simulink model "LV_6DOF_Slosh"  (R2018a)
settings: Solver=FixedStepAuto  StartTime=0.0  StopTime=489.8  FixedStep=0.0002  MaxStep=0.0001  RelTol=2e-6  EnableMultiTasking=on
InitFcn:
  | init
StopFcn:
  | pl
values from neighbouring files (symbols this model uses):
  accel = [97.3083,0,0]    [init.m]
  AcNoise = 0.1    [init.m]
  BBrcs = [82, 0.0, +3.375]    [init.m]
  Cdelay = 0.005    [init.m]
  Cza1 = FCS_Gains_Stg1(:, 5)    [init.m]
  d2r = pi/180    (= 0.0174532925199)    [init.m]    (also in pl.m; LQR_Design.m)
  Euler_0 = [90, 89.98, 0]*d2r    [init.m]
  fairing_mass = 1047.7*kg2slug    (= 71.7904994)    [init.m]
  Ie1 = 28.17    [init.m]
  Ie2 = 258.74    [init.m]
  Islosh = 1    [init.m]
  Isp = 65    [init.m]
  Ixxpr = Mass_Props(:,2)    [init.m]
  Ixypr = Mass_Props(:,5)    [init.m]
  Ixzpr = Mass_Props(:,6)    [init.m]
  Iyypr = Mass_Props(:,3)    [init.m]
  Iyzpr = Mass_Props(:,7)    [init.m]
  Izzpr = Mass_Props(:,4)    [init.m]
  Jdir = zeros(3,nt)    [init.m]
  JJ1 = Commands_2(:,2)    [init.m]
  JJ2 = Commands_2(:,3)    [init.m]
  JJ3 = Commands_2(:,4)    [init.m]
  Jloc = Jdir    [init.m]
  K_estim1 = FCS_Gains_Stg1(:,21)    [init.m]
  Kl_p1 = FCS_Gains_Stg1(:,12)    [init.m]
  Kl_phi1 = FCS_Gains_Stg1(:,11)    [init.m]
  Km_alfa1 = FCS_Gains_Stg1(:, 8)    [init.m]
  Km_alfin = FCS_Gains_Stg1(:,10)    [init.m]
  Km_q1 = FCS_Gains_Stg1(:, 7)    [init.m]
  Km_q2 = FCS_Gains_Stg2(:,5)    [init.m]
  Km_thet1 = FCS_Gains_Stg1(:, 6)    [init.m]
  Km_thet2 = FCS_Gains_Stg2(:,4)    [init.m]
  Km_thin1 = FCS_Gains_Stg1(:, 9)    [init.m]
  Km_thin2 = FCS_Gains_Stg2(:,6)    [init.m]
  Kmix2 = [ 0,   -1,    0;          0,    0,   -1]    [init.m]
  Kml1_1 = ee*FCS_Gains_Stg1(:,18)    [init.m]
  Kml2_1 = ee*FCS_Gains_Stg1(:,19)    [init.m]
  Kml2_2 = ee*FCS_Gains_Stg2(:,10)    [init.m]
  Kn_beta1 = FCS_Gains_Stg1(:,15)    [init.m]
  Kn_betin = FCS_Gains_Stg1(:,17)    [init.m]
  Kn_psi1 = FCS_Gains_Stg1(:,13)    [init.m]
  Kn_psi2 = FCS_Gains_Stg2(:,7)    [init.m]
  Kn_psin1 = FCS_Gains_Stg1(:,16)    [init.m]
  Kn_psin2 = FCS_Gains_Stg2(:,9)    [init.m]
  Kn_r1 = FCS_Gains_Stg1(:,14)    [init.m]
  Kn_r2 = FCS_Gains_Stg2(:,8)    [init.m]
  Le1 = 1.203    [init.m]
  Le2 = 2.892    [init.m]
  Massgn1 = ee*FCS_Gains_Stg1(:,2)    [init.m]
  Massgn2 = ee*FCS_Gains_Stg2(:,2)    [init.m]
  mdot1 = 2.5058    [init.m]
  mdot2 = 2.5058    [init.m]
  me1 = 9.325    [init.m]
  me2 = 13.927    [init.m]
  mrc = [x_ref, y_ref, z_ref]    [init.m]
  Msfue = Slosh(:,3)    [init.m]
  Mslox = Slosh(:,2)    [init.m]
  msspr = Mass_Props(:,1)    [init.m]
  Mvsls = Slosh(:,1)    [init.m]
  post_sep_wait = 4    [init.m]
  pre_sep_wait = 4    [init.m]
  Qbar1 = FCS_Gains_Stg1(:, 4)    [init.m]
  qtc1 = interp1(timi2(1:iend),Commands_2(1:iend, 9),timi2,'linear','extrap')    [init.m]
  qtc2 = interp1(timi2(1:iend),Commands_2(1:iend,10),timi2,'linear','extrap')    [init.m]
  qtc3 = interp1(timi2(1:iend),Commands_2(1:iend,11),timi2,'linear','extrap')    [init.m]
  qtc4 = interp1(timi2(1:iend),Commands_2(1:iend,12),timi2,'linear','extrap')    [init.m]
  r2d = 1/d2r    (= 57.2957795131)    [init.m]    (also in pl.m; LQR_Design.m)
  RBrcs = [82, +3.375, 0.0]    [init.m]
  Rfuel = Slosh(:,11)    [init.m]
  Rlox = Slosh(:,10)    [init.m]
  s1_dry_mass = 445.4969    [init.m]
  s1_init_prop_mass = 3.8002e+03    (= 3800.2)    [init.m]
  s2_dry_mass = 175.9451    [init.m]
  s2_init_prop_mass = 801.7606    [init.m]
  sp = 7.52    [init.m]
  Sref = 44.4146    [init.m]
  stage_to_fairing_sep_time = 34.7    [init.m]
  T3b = 176.6    [init.m]
  TBrcs = [82, 0.0, -3.375]    [init.m]
  thpnd = 15    [init.m]
  timi2 = Commands_2(:,1)    [init.m]
  TqLoad = 1    [init.m]
  tvc10 = [Xgmb2, 0.0,  0.0]    [init.m]
  tvc2 = [Xgmb1,  1.0202,  -2.4638]    [init.m]
  tvc3 = [Xgmb1, -1.0202,  -2.4638]    [init.m]
  tvc4 = [Xgmb1, -2.4638,  -1.0202]    [init.m]
  tvc5 = [Xgmb1, -2.4638,   1.0202]    [init.m]
  tvc6 = [Xgmb1, -1.0202,   2.4638]    [init.m]
  tvc7 = [Xgmb1,  1.0202,   2.4638]    [init.m]
  tvc8 = [Xgmb1,  2.4638,   1.0202]    [init.m]
  tvc9 = [Xgmb1,  0.0,      0.0]    [init.m]
  velpnd = 3    [init.m]
  Vrelgn1 = FCS_Gains_Stg1(:, 3)    [init.m]
  Vrelgn2 = FCS_Gains_Stg2(:,3)    [init.m]
  W_lowp1 = FCS_Gains_Stg1(:,22)    [init.m]
  W_nfilt1 = FCS_Gains_Stg1(:,20)    [init.m]
  Xcgpr = Mass_Props(:,8)    [init.m]
  Xfuel = Slosh(:,9)    [init.m]
  Xgmb1 = 10.7062    [init.m]
  Xgmb2 = 82.538    [init.m]
  Xlox = Slosh(:,8)    [init.m]
  Ycgpr = Mass_Props(:,9)    [init.m]
  Zcgpr = Mass_Props(:,10)    [init.m]
  Ztfue = Slosh(:,7)    [init.m]
  Ztlox = Slosh(:,6)    [init.m]
undefined symbols (not defined in the file or in its folder): Cl, Cl2, Cm, Cm2, Cn, Cn2, Continuous, cosd, CX, CX2, CY, CY2, CZ, CZ2, Dryden, Earth, F, ft, Isp1, Isp2, km, Kmix1, LBrcs, Light, MIL, q, r, sigbuilder_block, sind, STD, tvc1, WGS84
libraries: sharedutil x28, Actuator_Lib x18, simulink x4, aerolibasang x3, aerolibwind2 x3, sharedtransform x3, aerolibobsolete x2, aerolibconvert2 x2, aerolibatmos2 x1, aerolibadyn x1, aerolibutil x1
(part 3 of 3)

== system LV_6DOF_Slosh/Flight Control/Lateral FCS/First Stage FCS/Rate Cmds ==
  " " : Terminator
  Demux : Demux  Outputs=3
  Roll Rate Cmd : DiscretePulseGenerator  PulseType=Time based  Amplitude=10*d2r  Period=830  PhaseDelay=3.1  SampleTime=0.0002
  Sum1 : Sum  Inputs=-+|
  Transfer Fcn : TransferFcn  Denominator=[1 1]
  Pcm : Outport
  Rcm : Outport  Port=2
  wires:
  Demux/2 -> " "/1
  Demux/1 -> Sum1/2
  Sum1/1 -> Pcm/1
  [Gyros] -> Demux/1
  Demux/3 -> Rcm/1
  Roll Rate Cmd/1 -> Transfer Fcn/1
  Transfer Fcn/1 -> Sum1/1

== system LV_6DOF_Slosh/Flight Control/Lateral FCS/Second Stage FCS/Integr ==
  in : Inport
  Ground2 : Ground
  Switch : Switch  Criteria=u2 > Threshold
  int3 : Integrator
  ou : Outport
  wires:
  Ground2/1 -> Switch/3
  [s2_startup] -> Switch/2
  Switch/1 -> int3/1
  in/1 -> Switch/1
  int3/1 -> ou/1

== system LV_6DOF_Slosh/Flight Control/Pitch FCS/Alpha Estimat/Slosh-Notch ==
  note: Slosh Notch Filter
  In : Inport
  Ground : Ground
  Int1 : Integrator
  K_estim1 : Lookup  InputValues=Vrelgn1  Table=K_estim1
  Notch Filter : Subsystem
  Product1 : Product
  Switch1 : Switch  Criteria=u2 > Threshold
  Switch3 : Switch  Threshold=0.5
  Out : Outport
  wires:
  Product1/1 -> Int1/1
  Int1/1 -> Out/1
  [V0] -> K_estim1/1
  [Wnf] -> Switch3/2
  In/1 -> Switch1/3, Switch3/3
  Notch Filter/1(y) -> Switch3/1
  K_estim1/1 -> Product1/1
  [stage_sep] -> Switch1/2
  Ground/1 -> Switch1/1
  Switch1/1 -> Notch Filter/1(u)
  Switch3/1 -> Product1/2

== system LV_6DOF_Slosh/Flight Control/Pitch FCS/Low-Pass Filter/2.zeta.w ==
  in : Inport
  2.zet.w : Gain  Gain=1.25
  Product1 : Product
  ou : Outport
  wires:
  2.zet.w/1 -> Product1/1
  Product1/1 -> ou/1
  in/1 -> Product1/2
  [Wlp] -> 2.zet.w/1

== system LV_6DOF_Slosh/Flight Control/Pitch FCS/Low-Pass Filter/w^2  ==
  in : Inport
  Product : Product
  Product1 : Product
  ou : Outport
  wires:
  [Wlp] -> Product/1, Product/2
  Product/1 -> Product1/1
  Product1/1 -> ou/1
  in/1 -> Product1/2

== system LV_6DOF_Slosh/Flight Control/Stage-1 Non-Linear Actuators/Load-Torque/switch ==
  in : Inport
  Ground : Ground
  Ground1 : Ground
  Switch : Switch  Criteria=u2 > Threshold  Threshold=0.5
  Switch1 : Switch  Criteria=u2 > Threshold
  Torque Load Switch : Constant  Value=TqLoad
  ou : Outport
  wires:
  Torque Load Switch/1 -> Switch/2
  in/1 -> Switch/1
  Ground/1 -> Switch/3
  [s1_shutdown] -> Switch1/2
  Switch/1 -> Switch1/3
  Ground1/1 -> Switch1/1
  Switch1/1 -> ou/1

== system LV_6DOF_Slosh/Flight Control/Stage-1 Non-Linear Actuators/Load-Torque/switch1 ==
  in : Inport
  Ground : Ground
  Ground1 : Ground
  Switch : Switch  Criteria=u2 > Threshold  Threshold=0.5
  Switch1 : Switch  Criteria=u2 > Threshold
  Torque Load Switch : Constant  Value=TqLoad
  ou : Outport
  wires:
  Torque Load Switch/1 -> Switch/2
  in/1 -> Switch/1
  Ground/1 -> Switch/3
  [s1_shutdown] -> Switch1/2
  Switch/1 -> Switch1/3
  Ground1/1 -> Switch1/1
  Switch1/1 -> ou/1

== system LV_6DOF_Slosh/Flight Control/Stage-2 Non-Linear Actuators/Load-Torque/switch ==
  in : Inport
  Ground : Ground
  Ground1 : Ground
  Switch : Switch  Criteria=u2 > Threshold  Threshold=0.5
  Switch1 : Switch  Criteria=u2 > Threshold
  Torque Load Switch : Constant  Value=TqLoad
  ou : Outport
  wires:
  Torque Load Switch/1 -> Switch/2
  in/1 -> Switch/1
  Ground/1 -> Switch/3
  Switch1/1 -> ou/1
  Switch/1 -> Switch1/1
  Ground1/1 -> Switch1/3
  [s2_startup] -> Switch1/2

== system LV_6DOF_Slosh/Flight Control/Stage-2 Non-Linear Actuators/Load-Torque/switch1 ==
  in : Inport
  Ground : Ground
  Ground1 : Ground
  Switch : Switch  Criteria=u2 > Threshold  Threshold=0.5
  Switch1 : Switch  Criteria=u2 > Threshold
  Torque Load Switch : Constant  Value=TqLoad
  ou : Outport
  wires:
  Torque Load Switch/1 -> Switch/2
  in/1 -> Switch/1
  Ground/1 -> Switch/3
  Switch1/1 -> ou/1
  Switch/1 -> Switch1/1
  Ground1/1 -> Switch1/3
  [s2_startup] -> Switch1/2

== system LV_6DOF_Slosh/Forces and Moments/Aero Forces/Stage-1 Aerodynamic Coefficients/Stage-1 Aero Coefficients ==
  note: Stage-1 Aero
  albet : Inport
  Mach : Inport  Port=2
  Alpha Lookup : PreLookup  BreakpointsData=Alfa1  BeginIndexSearchUsingPreviousIndexResult=on  ExtrapMethod=Linear
  Beta Lookup : PreLookup  BreakpointsData=Beta1  BeginIndexSearchUsingPreviousIndexResult=on  ExtrapMethod=Linear
  CX : Interpolation_n-D  NumberOfTableDimensions=3  Table=CX  RemoveProtectionIndex=on
  CY : Interpolation_n-D  NumberOfTableDimensions=3  Table=CY  RemoveProtectionIndex=on
  CZ : Interpolation_n-D  NumberOfTableDimensions=3  Table=CZ  RemoveProtectionIndex=on
  Cl : Interpolation_n-D  NumberOfTableDimensions=3  Table=Cl  RemoveProtectionIndex=on  OutDataTypeStr=double
  Cm : Interpolation_n-D  NumberOfTableDimensions=3  Table=Cm  RemoveProtectionIndex=on
  Cn : Interpolation_n-D  NumberOfTableDimensions=3  Table=Cn  RemoveProtectionIndex=on
  Demux : Demux  Outputs=2
  Mach Lookup : PreLookup  BreakpointsData=Mach1  BeginIndexSearchUsingPreviousIndexResult=on  ExtrapMethod=Linear
  Mux1 : Mux  Inputs=6
  Coeff : Outport  InitialOutput=0
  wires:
  Mux1/1 -> Coeff/1
  Mach/1 -> Mach Lookup/1
  albet/1 -> Demux/1
  Demux/2 -> Beta Lookup/1
  Beta Lookup/2 -> CZ/6, Cl/6, Cn/6, Cm/6, CY/6, CX/6
  Beta Lookup/1 -> CY/5, CZ/5, Cl/5, Cn/5, Cm/5, CX/5
  Mach Lookup/2 -> CX/4, CZ/4, Cl/4, Cn/4, Cm/4, CY/4
  Mach Lookup/1 -> CX/3, CZ/3, Cl/3, Cn/3, Cm/3, CY/3
  Alpha Lookup/2 -> Cn/2, Cm/2, Cl/2, CZ/2, CY/2, CX/2
  Alpha Lookup/1 -> CZ/1, Cl/1, Cn/1, Cm/1, CY/1, CX/1
  Cn/1 -> Mux1/6
  Cm/1 -> Mux1/5
  Cl/1 -> Mux1/4
  CZ/1 -> Mux1/3
  CY/1 -> Mux1/2
  CX/1 -> Mux1/1
  Demux/1 -> Alpha Lookup/1

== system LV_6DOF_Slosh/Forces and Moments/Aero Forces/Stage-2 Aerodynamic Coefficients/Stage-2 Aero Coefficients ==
  note: Stage-2 Aero
  albet : Inport
  Mach : Inport  Port=2
  Alpha Lookup : PreLookup  BreakpointsData=Alfa2  BeginIndexSearchUsingPreviousIndexResult=on  ExtrapMethod=Linear
  Beta Lookup : PreLookup  BreakpointsData=Beta2  BeginIndexSearchUsingPreviousIndexResult=on  ExtrapMethod=Linear
  CX2 : Interpolation_n-D  NumberOfTableDimensions=3  Table=CX2  RemoveProtectionIndex=on
  CY2 : Interpolation_n-D  NumberOfTableDimensions=3  Table=CY2  RemoveProtectionIndex=on
  CZ2 : Interpolation_n-D  NumberOfTableDimensions=3  Table=CZ2  RemoveProtectionIndex=on
  Cl2 : Interpolation_n-D  NumberOfTableDimensions=3  Table=Cl2  RemoveProtectionIndex=on  OutDataTypeStr=double
  Cm2 : Interpolation_n-D  NumberOfTableDimensions=3  Table=Cm2  RemoveProtectionIndex=on
  Cn2 : Interpolation_n-D  NumberOfTableDimensions=3  Table=Cn2  RemoveProtectionIndex=on
  Demux : Demux  Outputs=2
  Mach Lookup : PreLookup  BreakpointsData=Mach2  BeginIndexSearchUsingPreviousIndexResult=on  ExtrapMethod=Linear
  Mux1 : Mux  Inputs=6
  Coeff : Outport  InitialOutput=0
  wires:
  Mux1/1 -> Coeff/1
  Mach/1 -> Mach Lookup/1
  albet/1 -> Demux/1
  Demux/2 -> Beta Lookup/1
  Beta Lookup/2 -> CZ2/6, Cl2/6, Cn2/6, Cm2/6, CY2/6, CX2/6
  Beta Lookup/1 -> CY2/5, CZ2/5, Cl2/5, Cn2/5, Cm2/5, CX2/5
  Mach Lookup/2 -> CX2/4, CZ2/4, Cl2/4, Cn2/4, Cm2/4, CY2/4
  Mach Lookup/1 -> CX2/3, CZ2/3, Cl2/3, Cn2/3, Cm2/3, CY2/3
  Alpha Lookup/2 -> Cn2/2, Cm2/2, Cl2/2, CZ2/2, CY2/2, CX2/2
  Alpha Lookup/1 -> CZ2/1, Cl2/1, Cn2/1, Cm2/1, CY2/1, CX2/1
  Cn2/1 -> Mux1/6
  Cm2/1 -> Mux1/5
  Cl2/1 -> Mux1/4
  CZ2/1 -> Mux1/3
  CY2/1 -> Mux1/2
  Demux/1 -> Alpha Lookup/1
  CX2/1 -> Mux1/1

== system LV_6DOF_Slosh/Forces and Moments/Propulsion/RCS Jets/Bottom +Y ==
  f(2) : Inport
  3x3 Cross Product3 : sharedutil/3x3 Cross Product  aMode=aMode
  Bottom +Y RCS : Subsystem
  T2 : Outport
  F2 : Outport  Port=2
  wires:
  [BBrln] -> 3x3 Cross Product3/1
  3x3 Cross Product3/1 -> T2/1
  f(2)/1 -> Bottom +Y RCS/1(Thrust)
  Bottom +Y RCS/1(FL) -> F2/1, 3x3 Cross Product3/2

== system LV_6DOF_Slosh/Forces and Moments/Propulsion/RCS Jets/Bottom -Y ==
  f(4) : Inport
  3x3 Cross Product3 : sharedutil/3x3 Cross Product  aMode=aMode
  Bottom -Y RCS : Subsystem
  T4 : Outport
  F4 : Outport  Port=2
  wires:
  [BBrln] -> 3x3 Cross Product3/1
  3x3 Cross Product3/1 -> T4/1
  f(4)/1 -> Bottom -Y RCS/1(Thrust)
  Bottom -Y RCS/1(FL) -> F4/1, 3x3 Cross Product3/2

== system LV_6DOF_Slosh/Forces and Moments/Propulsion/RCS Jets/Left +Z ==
  f(5) : Inport
  3x3 Cross Product3 : sharedutil/3x3 Cross Product  aMode=aMode
  Left +Z RCS : Subsystem
  T5 : Outport
  F5 : Outport  Port=2
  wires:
  [LBrln] -> 3x3 Cross Product3/1
  3x3 Cross Product3/1 -> T5/1
  f(5)/1 -> Left +Z RCS/1(Thrust)
  Left +Z RCS/1(FL) -> F5/1, 3x3 Cross Product3/2

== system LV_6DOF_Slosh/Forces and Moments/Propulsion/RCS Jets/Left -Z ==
  f(7) : Inport
  3x3 Cross Product5 : sharedutil/3x3 Cross Product  aMode=aMode
  "Left, -Z RCS" : Subsystem
  T7 : Outport
  F7 : Outport  Port=2
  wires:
  3x3 Cross Product5/1 -> T7/1
  "Left, -Z RCS"/1(FL) -> F7/1, 3x3 Cross Product5/2
  [LBrln] -> 3x3 Cross Product5/1
  f(7)/1 -> "Left, -Z RCS"/1(Thrust)

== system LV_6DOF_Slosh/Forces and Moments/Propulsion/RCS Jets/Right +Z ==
  f(6) : Inport
  3x3 Cross Product3 : sharedutil/3x3 Cross Product  aMode=aMode
  Right +Z RCS : Subsystem
  T6 : Outport
  F6 : Outport  Port=2
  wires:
  [RBrln] -> 3x3 Cross Product3/1
  3x3 Cross Product3/1 -> T6/1
  f(6)/1 -> Right +Z RCS/1(Thrust)
  Right +Z RCS/1(FL) -> F6/1, 3x3 Cross Product3/2

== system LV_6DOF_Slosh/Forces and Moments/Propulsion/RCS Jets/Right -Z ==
  f(8) : Inport
  3x3 Cross Product5 : sharedutil/3x3 Cross Product  aMode=aMode
  Right -Z RCS : Subsystem
  T8 : Outport
  F8 : Outport  Port=2
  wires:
  3x3 Cross Product5/1 -> T8/1
  Right -Z RCS/1(FL) -> F8/1, 3x3 Cross Product5/2
  [RBrln] -> 3x3 Cross Product5/1
  f(8)/1 -> Right -Z RCS/1(Thrust)

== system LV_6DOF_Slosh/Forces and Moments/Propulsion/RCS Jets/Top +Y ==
  f(1) : Inport
  3x3 Cross Product3 : sharedutil/3x3 Cross Product  aMode=aMode
  Top +Y RCS : Subsystem
  T1 : Outport
  F1 : Outport  Port=2
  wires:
  [TBrln] -> 3x3 Cross Product3/1
  3x3 Cross Product3/1 -> T1/1
  f(1)/1 -> Top +Y RCS/1(Thrust)
  Top +Y RCS/1(FL) -> F1/1, 3x3 Cross Product3/2

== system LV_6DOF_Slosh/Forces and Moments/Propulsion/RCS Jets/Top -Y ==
  f(3) : Inport
  3x3 Cross Product3 : sharedutil/3x3 Cross Product  aMode=aMode
  Top -Y RCS : Subsystem
  T3 : Outport
  F3 : Outport  Port=2
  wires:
  [TBrln] -> 3x3 Cross Product3/1
  3x3 Cross Product3/1 -> T3/1
  f(3)/1 -> Top -Y RCS/1(Thrust)
  Top -Y RCS/1(FL) -> F3/1, 3x3 Cross Product3/2

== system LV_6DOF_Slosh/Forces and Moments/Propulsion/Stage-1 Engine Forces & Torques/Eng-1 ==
  note: Engine #1 Force
  Thrust : Inport
  dy : Inport  Port=2
  dz : Inport  Port=3
  -1 : Gain  Gain=-1
  1/9 : Gain  Gain=1/9
  3x3 Cross Product : sharedutil/3x3 Cross Product  aMode=aMode
  Fx1 : Product  Inputs=3
  Fy1 : Product  Inputs=3
  Fz1 : Product
  Mux : Mux  Inputs=3
  cos(dy) : Trigonometry  Operator=cos
  cos(dz) : Trigonometry  Operator=cos
  sin(dy) : Trigonometry
  sin(dz) : Trigonometry
  F1 : Outport  InitialOutput=0
  M1 : Outport  Port=2  InitialOutput=0
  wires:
  dz/1 -> sin(dz)/1, cos(dz)/1
  dy/1 -> sin(dy)/1, cos(dy)/1
  sin(dy)/1 -> Fz1/2
  sin(dz)/1 -> Fy1/3
  cos(dz)/1 -> Fx1/3
  Mux/1 -> 3x3 Cross Product/2, F1/1
  Fx1/1 -> Mux/1
  Fz1/1 -> Mux/3
  Fy1/1 -> Mux/2
  -1/1 -> Fz1/1
  cos(dy)/1 -> Fx1/2, Fy1/2
  Thrust/1 -> 1/9/1
  [lg1] -> 3x3 Cross Product/1
  3x3 Cross Product/1 -> M1/1
  1/9/1 -> -1/1, Fx1/1, Fy1/1

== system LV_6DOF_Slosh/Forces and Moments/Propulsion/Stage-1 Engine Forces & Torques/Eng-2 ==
  note: Engine #2 Force
  Thrust : Inport
  dy : Inport  Port=2
  dz : Inport  Port=3
  -1 : Gain  Gain=-1
  1/9 : Gain  Gain=1/9
  3x3 Cross Product : sharedutil/3x3 Cross Product  aMode=aMode
  Fx2 : Product  Inputs=3
  Fy2 : Product  Inputs=3
  Fz2 : Product
  Mux : Mux  Inputs=3
  cos(dy) : Trigonometry  Operator=cos
  cos(dz) : Trigonometry  Operator=cos
  sin(dy) : Trigonometry
  sin(dz) : Trigonometry
  F2 : Outport  InitialOutput=0
  M2 : Outport  Port=2  InitialOutput=0
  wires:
  dz/1 -> sin(dz)/1, cos(dz)/1
  dy/1 -> sin(dy)/1, cos(dy)/1
  sin(dy)/1 -> Fz2/2
  sin(dz)/1 -> Fy2/3
  cos(dz)/1 -> Fx2/3
  Mux/1 -> 3x3 Cross Product/2, F2/1
  Fx2/1 -> Mux/1
  Fz2/1 -> Mux/3
  Fy2/1 -> Mux/2
  -1/1 -> Fz2/1
  cos(dy)/1 -> Fx2/2, Fy2/2
  Thrust/1 -> 1/9/1
  [lg2] -> 3x3 Cross Product/1
  3x3 Cross Product/1 -> M2/1
  1/9/1 -> -1/1, Fx2/1, Fy2/1

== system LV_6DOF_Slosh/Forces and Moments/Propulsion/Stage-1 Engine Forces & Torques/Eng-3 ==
  note: Engine #3 Force
  Thrust : Inport
  dy : Inport  Port=2
  dz : Inport  Port=3
  -1 : Gain  Gain=-1
  1/9 : Gain  Gain=1/9
  3x3 Cross Product : sharedutil/3x3 Cross Product  aMode=aMode
  Fx3 : Product  Inputs=3
  Fy3 : Product  Inputs=3
  Fz3 : Product
  Mux : Mux  Inputs=3
  cos(dy) : Trigonometry  Operator=cos
  cos(dz) : Trigonometry  Operator=cos
  sin(dy) : Trigonometry
  sin(dz) : Trigonometry
  F3 : Outport  InitialOutput=0
  M3 : Outport  Port=2  InitialOutput=0
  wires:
  dz/1 -> sin(dz)/1, cos(dz)/1
  dy/1 -> sin(dy)/1, cos(dy)/1
  sin(dy)/1 -> Fz3/2
  sin(dz)/1 -> Fy3/3
  cos(dz)/1 -> Fx3/3
  Mux/1 -> 3x3 Cross Product/2, F3/1
  Fx3/1 -> Mux/1
  Fz3/1 -> Mux/3
  Fy3/1 -> Mux/2
  -1/1 -> Fz3/1
  cos(dy)/1 -> Fx3/2, Fy3/2
  Thrust/1 -> 1/9/1
  [lg3] -> 3x3 Cross Product/1
  3x3 Cross Product/1 -> M3/1
  1/9/1 -> -1/1, Fx3/1, Fy3/1

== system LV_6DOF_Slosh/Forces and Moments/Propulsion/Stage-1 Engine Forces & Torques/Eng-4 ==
  note: Engine #4 Force
  Thrust : Inport
  dy : Inport  Port=2
  dz : Inport  Port=3
  -1 : Gain  Gain=-1
  1/9 : Gain  Gain=1/9
  3x3 Cross Product : sharedutil/3x3 Cross Product  aMode=aMode
  Fx4 : Product  Inputs=3
  Fy4 : Product  Inputs=3
  Fz4 : Product
  Mux : Mux  Inputs=3
  cos(dy) : Trigonometry  Operator=cos
  cos(dz) : Trigonometry  Operator=cos
  sin(dy) : Trigonometry
  sin(dz) : Trigonometry
  F4 : Outport  InitialOutput=0
  M4 : Outport  Port=2  InitialOutput=0
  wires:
  dz/1 -> sin(dz)/1, cos(dz)/1
  dy/1 -> sin(dy)/1, cos(dy)/1
  sin(dy)/1 -> Fz4/2
  sin(dz)/1 -> Fy4/3
  cos(dz)/1 -> Fx4/3
  Mux/1 -> 3x3 Cross Product/2, F4/1
  Fx4/1 -> Mux/1
  Fz4/1 -> Mux/3
  Fy4/1 -> Mux/2
  -1/1 -> Fz4/1
  cos(dy)/1 -> Fx4/2, Fy4/2
  Thrust/1 -> 1/9/1
  [lg4] -> 3x3 Cross Product/1
  3x3 Cross Product/1 -> M4/1
  1/9/1 -> -1/1, Fx4/1, Fy4/1

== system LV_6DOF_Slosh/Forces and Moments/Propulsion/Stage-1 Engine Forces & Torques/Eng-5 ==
  note: Engine #5 Force
  Thrust : Inport
  dy : Inport  Port=2
  dz : Inport  Port=3
  -1 : Gain  Gain=-1
  1/9 : Gain  Gain=1/9
  3x3 Cross Product : sharedutil/3x3 Cross Product  aMode=aMode
  Fx5 : Product  Inputs=3
  Fy5 : Product  Inputs=3
  Fz5 : Product
  Mux : Mux  Inputs=3
  cos(dy) : Trigonometry  Operator=cos
  cos(dz) : Trigonometry  Operator=cos
  sin(dy) : Trigonometry
  sin(dz) : Trigonometry
  F5 : Outport  InitialOutput=0
  M5 : Outport  Port=2  InitialOutput=0
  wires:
  dz/1 -> sin(dz)/1, cos(dz)/1
  dy/1 -> sin(dy)/1, cos(dy)/1
  sin(dy)/1 -> Fz5/2
  sin(dz)/1 -> Fy5/3
  cos(dz)/1 -> Fx5/3
  Mux/1 -> 3x3 Cross Product/2, F5/1
  Fx5/1 -> Mux/1
  Fz5/1 -> Mux/3
  Fy5/1 -> Mux/2
  -1/1 -> Fz5/1
  cos(dy)/1 -> Fx5/2, Fy5/2
  Thrust/1 -> 1/9/1
  [lg5] -> 3x3 Cross Product/1
  3x3 Cross Product/1 -> M5/1
  1/9/1 -> -1/1, Fx5/1, Fy5/1

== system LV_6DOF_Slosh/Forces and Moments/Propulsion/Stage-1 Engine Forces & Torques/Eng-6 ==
  note: Engine #6 Force
  Thrust : Inport
  dy : Inport  Port=2
  dz : Inport  Port=3
  -1 : Gain  Gain=-1
  1/9 : Gain  Gain=1/9
  3x3 Cross Product : sharedutil/3x3 Cross Product  aMode=aMode
  Fx6 : Product  Inputs=3
  Fy6 : Product  Inputs=3
  Fz6 : Product
  Mux : Mux  Inputs=3
  cos(dy) : Trigonometry  Operator=cos
  cos(dz) : Trigonometry  Operator=cos
  sin(dy) : Trigonometry
  sin(dz) : Trigonometry
  F6 : Outport  InitialOutput=0
  M6 : Outport  Port=2  InitialOutput=0
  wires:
  dz/1 -> sin(dz)/1, cos(dz)/1
  dy/1 -> sin(dy)/1, cos(dy)/1
  sin(dy)/1 -> Fz6/2
  sin(dz)/1 -> Fy6/3
  cos(dz)/1 -> Fx6/3
  Mux/1 -> 3x3 Cross Product/2, F6/1
  Fx6/1 -> Mux/1
  Fz6/1 -> Mux/3
  Fy6/1 -> Mux/2
  -1/1 -> Fz6/1
  cos(dy)/1 -> Fx6/2, Fy6/2
  Thrust/1 -> 1/9/1
  [lg6] -> 3x3 Cross Product/1
  3x3 Cross Product/1 -> M6/1
  1/9/1 -> -1/1, Fx6/1, Fy6/1

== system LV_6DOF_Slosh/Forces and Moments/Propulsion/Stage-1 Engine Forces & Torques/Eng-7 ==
  note: Engine #7 Force
  Thrust : Inport
  dy : Inport  Port=2
  dz : Inport  Port=3
  -1 : Gain  Gain=-1
  1/9 : Gain  Gain=1/9
  3x3 Cross Product : sharedutil/3x3 Cross Product  aMode=aMode
  Fx7 : Product  Inputs=3
  Fy7 : Product  Inputs=3
  Fz7 : Product
  Mux : Mux  Inputs=3
  cos(dy) : Trigonometry  Operator=cos
  cos(dz) : Trigonometry  Operator=cos
  sin(dy) : Trigonometry
  sin(dz) : Trigonometry
  F7 : Outport  InitialOutput=0
  M7 : Outport  Port=2  InitialOutput=0
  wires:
  dz/1 -> sin(dz)/1, cos(dz)/1
  dy/1 -> sin(dy)/1, cos(dy)/1
  sin(dy)/1 -> Fz7/2
  sin(dz)/1 -> Fy7/3
  cos(dz)/1 -> Fx7/3
  Mux/1 -> F7/1, 3x3 Cross Product/2
  Fx7/1 -> Mux/1
  Fz7/1 -> Mux/3
  Fy7/1 -> Mux/2
  -1/1 -> Fz7/1
  cos(dy)/1 -> Fx7/2, Fy7/2
  Thrust/1 -> 1/9/1
  [lg7] -> 3x3 Cross Product/1
  3x3 Cross Product/1 -> M7/1
  1/9/1 -> -1/1, Fx7/1, Fy7/1

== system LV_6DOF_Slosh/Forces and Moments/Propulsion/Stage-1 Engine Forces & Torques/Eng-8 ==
  note: Engine #8 Force
  Thrust : Inport
  dy : Inport  Port=2
  dz : Inport  Port=3
  -1 : Gain  Gain=-1
  1/9 : Gain  Gain=1/9
  3x3 Cross Product : sharedutil/3x3 Cross Product  aMode=aMode
  Fx8 : Product  Inputs=3
  Fy8 : Product  Inputs=3
  Fz8 : Product
  Mux : Mux  Inputs=3
  cos(dy) : Trigonometry  Operator=cos
  cos(dz) : Trigonometry  Operator=cos
  sin(dy) : Trigonometry
  sin(dz) : Trigonometry
  F8 : Outport  InitialOutput=0
  M8 : Outport  Port=2  InitialOutput=0
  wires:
  dz/1 -> sin(dz)/1, cos(dz)/1
  dy/1 -> sin(dy)/1, cos(dy)/1
  sin(dy)/1 -> Fz8/2
  sin(dz)/1 -> Fy8/3
  cos(dz)/1 -> Fx8/3
  Mux/1 -> 3x3 Cross Product/2, F8/1
  Fx8/1 -> Mux/1
  Fz8/1 -> Mux/3
  Fy8/1 -> Mux/2
  -1/1 -> Fz8/1
  cos(dy)/1 -> Fx8/2, Fy8/2
  Thrust/1 -> 1/9/1
  [lg8] -> 3x3 Cross Product/1
  3x3 Cross Product/1 -> M8/1
  1/9/1 -> -1/1, Fx8/1, Fy8/1

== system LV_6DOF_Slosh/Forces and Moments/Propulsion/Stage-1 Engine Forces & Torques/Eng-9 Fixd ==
  note: Fixed Engine #9 Force
  Thrust : Inport
  1/9 : Gain  Gain=1/9
  3x3 Cross Product : sharedutil/3x3 Cross Product  aMode=aMode
  Ground : Ground
  Mux : Mux  Inputs=3
  F9 : Outport  InitialOutput=0
  M9 : Outport  Port=2  InitialOutput=0
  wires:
  Mux/1 -> 3x3 Cross Product/2, F9/1
  Ground/1 -> Mux/3, Mux/2
  Thrust/1 -> 1/9/1
  [lg9] -> 3x3 Cross Product/1
  3x3 Cross Product/1 -> M9/1
  1/9/1 -> Mux/1  "FX9"

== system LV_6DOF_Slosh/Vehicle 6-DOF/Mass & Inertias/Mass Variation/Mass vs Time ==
  Demux : Demux  Tag=STV Demux  Outputs=1
  FromWs : FromWorkspace  Tag=STV FromWs  VariableName=tuvar  SampleTime=0
  Mass (slg) : Outport  Tag=STV Outport
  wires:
  FromWs/1 -> Demux/1
  Demux/1 -> Mass (slg)/1

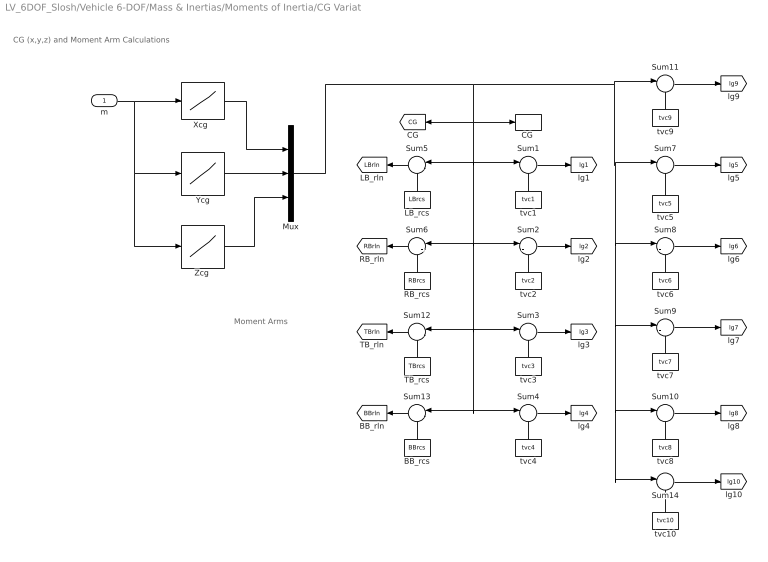
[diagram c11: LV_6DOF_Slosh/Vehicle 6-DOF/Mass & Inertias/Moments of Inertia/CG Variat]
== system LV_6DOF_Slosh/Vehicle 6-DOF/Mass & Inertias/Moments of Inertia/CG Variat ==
  note: Moment Arms
  note: CG (x,y,z) and Moment Arm Calculations
  m : Inport
  BB_rcs : Constant  Value=BBrcs
  "CG " : ToWorkspace  VariableName=CG  SampleTime=-1
  LB_rcs : Constant  Value=LBrcs
  Mux : Mux  Inputs=3
  RB_rcs : Constant  Value=RBrcs
  Sum{1..14} (14 alike) : Sum  Inputs=|-+
  TB_rcs : Constant  Value=TBrcs
  "Xcg  " : Lookup  InputValues=msspr  Table=Xcgpr
  Ycg : Lookup  InputValues=msspr  Table=Ycgpr
  "Zcg " : Lookup  InputValues=msspr  Table=Zcgpr
  tvc1 : Constant  Value=tvc1
  tvc10 : Constant  Value=tvc10
  tvc2 : Constant  Value=tvc2
  tvc3 : Constant  Value=tvc3
  tvc4 : Constant  Value=tvc4
  tvc5 : Constant  Value=tvc5
  tvc6 : Constant  Value=tvc6
  tvc7 : Constant  Value=tvc7
  tvc8 : Constant  Value=tvc8
  tvc9 : Constant  Value=tvc9
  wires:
  Sum14/1 -> [lg10]
  tvc10/1 -> Sum14/2
  Sum5/1 -> [LBrln]
  Sum6/1 -> [RBrln]
  tvc7/1 -> Sum9/2
  tvc8/1 -> Sum10/2
  tvc9/1 -> Sum11/2
  tvc6/1 -> Sum8/2
  tvc5/1 -> Sum7/2
  Sum11/1 -> [lg9]
  Sum10/1 -> [lg8]
  Sum9/1 -> [lg7]
  Sum8/1 -> [lg6]
  Sum7/1 -> [lg5]
  RB_rcs/1 -> Sum6/2
  LB_rcs/1 -> Sum5/2
  Sum4/1 -> [lg4]
  tvc4/1 -> Sum4/2
  Sum3/1 -> [lg3]
  tvc3/1 -> Sum3/2
  Sum2/1 -> [lg2]
  tvc2/1 -> Sum2/2
  tvc1/1 -> Sum1/2
  Sum1/1 -> [lg1]
  Mux/1 -> Sum11/1, Sum7/1, Sum8/1, Sum9/1, Sum14/1, Sum10/1, Sum13/1, Sum4/1, Sum12/1, Sum3/1, Sum2/1, Sum6/1, Sum1/1, Sum5/1, "CG "/1, [CG]
  "Xcg  "/1 -> Mux/1
  "Zcg "/1 -> Mux/3
  Ycg/1 -> Mux/2
  m/1 -> "Zcg "/1, Ycg/1, "Xcg  "/1
  TB_rcs/1 -> Sum12/2
  BB_rcs/1 -> Sum13/2
  Sum12/1 -> [TBrln]
  Sum13/1 -> [BBrln]

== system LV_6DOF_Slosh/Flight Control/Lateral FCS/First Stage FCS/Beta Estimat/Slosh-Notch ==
  In : Inport
  Ground : Ground
  Int1 : Integrator
  K_estim1 : Lookup  InputValues=Vrelgn1  Table=K_estim1
  Notch Filter : Subsystem
  Product1 : Product
  Switch1 : Switch  Criteria=u2 > Threshold
  Switch3 : Switch  Threshold=0.5
  Out : Outport
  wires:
  Product1/1 -> Int1/1
  Switch3/1 -> Product1/2
  Int1/1 -> Out/1
  [V0] -> K_estim1/1
  [Wnf] -> Switch3/2
  Notch Filter/1(y) -> Switch3/1
  K_estim1/1 -> Product1/1
  [stage_sep] -> Switch1/2
  Ground/1 -> Switch1/1
  Switch1/1 -> Notch Filter/1(u)
  In/1 -> Switch3/3, Switch1/3

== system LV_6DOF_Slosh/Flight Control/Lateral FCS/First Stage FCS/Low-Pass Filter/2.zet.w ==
  in : Inport
  2.zet.w : Gain  Gain=1.25
  Product1 : Product
  ou : Outport
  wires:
  2.zet.w/1 -> Product1/1
  Product1/1 -> ou/1
  in/1 -> Product1/2
  [Wlp] -> 2.zet.w/1

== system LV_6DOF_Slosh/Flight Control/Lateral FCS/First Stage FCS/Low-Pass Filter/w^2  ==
  in : Inport
  Product : Product
  Product1 : Product
  ou : Outport
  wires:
  [Wlp] -> Product/1, Product/2
  Product/1 -> Product1/1
  Product1/1 -> ou/1
  in/1 -> Product1/2

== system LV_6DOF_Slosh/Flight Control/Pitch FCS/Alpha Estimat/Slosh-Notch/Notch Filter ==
  note: Variable Notch Filter
  note: Notch Frequency Varies with V-relative
  u : Inport
  2.z1.w : Subsystem
  2.z2.w : Subsystem
  Constant : Constant
  Sum1 : Sum  Inputs=+++
  Sum3 : Sum  Inputs=+--
  Switch1 : Switch  Criteria=u2 > Threshold
  W_nfilt1 : Lookup  InputValues=Vrelgn1  Table=W_nfilt1
  int{1..4} (4 alike) : Integrator
  w^2 : Subsystem
  "w^2 " : Subsystem
  y : Outport
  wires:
  u/1 -> Sum1/1, int1/1
  int2/1 -> "w^2 "/1(in)
  int1/1 -> 2.z1.w/1(in), int2/1
  int3/1 -> 2.z2.w/1(in), int4/1
  Sum1/1 -> Sum3/1
  Sum3/1 -> y/1, int3/1
  2.z2.w/1(ou) -> Sum3/3
  int4/1 -> w^2/1(in)
  "w^2 "/1(ou) -> Sum1/3
  w^2/1(ou) -> Sum3/2
  2.z1.w/1(ou) -> Sum1/2
  [V0] -> W_nfilt1/1
  [stage_sep] -> Switch1/2
  Switch1/1 -> [Wnf]
  Constant/1 -> Switch1/1
  W_nfilt1/1 -> Switch1/3

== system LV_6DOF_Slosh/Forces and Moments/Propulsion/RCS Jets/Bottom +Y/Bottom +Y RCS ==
  note: Bottom, +Y RCS Force
  Thrust : Inport
  -1 : Gain  Gain=-1
  Fx1 : Product  Inputs=3
  Fy1 : Product  Inputs=3
  Fz1 : Product
  Mux : Mux  Inputs=3
  cos(dy) : Trigonometry  Operator=cos
  cos(dz) : Trigonometry  Operator=cos
  dy=0 : Constant  Value=0
  dz=+90 : Constant  Value=+90*d2r
  sin(dy) : Trigonometry
  sin(dz) : Trigonometry
  FL : Outport  InitialOutput=0
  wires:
  dz=+90/1 -> sin(dz)/1, cos(dz)/1
  dy=0/1 -> sin(dy)/1, cos(dy)/1
  sin(dy)/1 -> Fz1/2
  sin(dz)/1 -> Fy1/3
  cos(dz)/1 -> Fx1/3
  Mux/1 -> FL/1
  Fx1/1 -> Mux/1
  Fz1/1 -> Mux/3
  Fy1/1 -> Mux/2
  -1/1 -> Fz1/1
  cos(dy)/1 -> Fx1/2, Fy1/2
  Thrust/1 -> Fx1/1, Fy1/1, -1/1

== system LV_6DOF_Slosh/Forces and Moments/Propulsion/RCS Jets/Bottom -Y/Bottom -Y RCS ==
  note: Bottom -Y RCS Force
  Thrust : Inport
  -1 : Gain  Gain=-1
  Fx1 : Product  Inputs=3
  Fy1 : Product  Inputs=3
  Fz1 : Product
  Mux : Mux  Inputs=3
  cos(dy) : Trigonometry  Operator=cos
  cos(dz) : Trigonometry  Operator=cos
  dy=0 : Constant  Value=0
  dz=-90 : Constant  Value=-90*d2r
  sin(dy) : Trigonometry
  sin(dz) : Trigonometry
  FL : Outport  InitialOutput=0
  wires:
  dz=-90/1 -> sin(dz)/1, cos(dz)/1
  dy=0/1 -> sin(dy)/1, cos(dy)/1
  sin(dy)/1 -> Fz1/2
  sin(dz)/1 -> Fy1/3
  cos(dz)/1 -> Fx1/3
  Mux/1 -> FL/1
  Fx1/1 -> Mux/1
  Fz1/1 -> Mux/3
  Fy1/1 -> Mux/2
  -1/1 -> Fz1/1
  cos(dy)/1 -> Fx1/2, Fy1/2
  Thrust/1 -> Fx1/1, Fy1/1, -1/1

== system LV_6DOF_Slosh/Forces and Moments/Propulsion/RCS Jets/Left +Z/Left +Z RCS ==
  note: Left +Z RCS Force
  Thrust : Inport
  -1 : Gain  Gain=-1
  Fx1 : Product  Inputs=3
  Fy1 : Product  Inputs=3
  Fz1 : Product
  Mux : Mux  Inputs=3
  cos(dy) : Trigonometry  Operator=cos
  cos(dz) : Trigonometry  Operator=cos
  dy=-90 : Constant  Value=-90*d2r
  dz=0 : Constant  Value=0
  sin(dy) : Trigonometry
  sin(dz) : Trigonometry
  FL : Outport  InitialOutput=0
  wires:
  dz=0/1 -> sin(dz)/1, cos(dz)/1
  dy=-90/1 -> sin(dy)/1, cos(dy)/1
  sin(dy)/1 -> Fz1/2
  sin(dz)/1 -> Fy1/3
  cos(dz)/1 -> Fx1/3
  Mux/1 -> FL/1
  Fx1/1 -> Mux/1
  Fz1/1 -> Mux/3
  Fy1/1 -> Mux/2
  -1/1 -> Fz1/1
  cos(dy)/1 -> Fx1/2, Fy1/2
  Thrust/1 -> Fx1/1, Fy1/1, -1/1

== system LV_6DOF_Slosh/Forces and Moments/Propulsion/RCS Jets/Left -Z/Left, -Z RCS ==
  note: Left -Z RCS Force
  Thrust : Inport
  -1 : Gain  Gain=-1
  Fx1 : Product  Inputs=3
  Fy1 : Product  Inputs=3
  Fz1 : Product
  Mux : Mux  Inputs=3
  cos(dy) : Trigonometry  Operator=cos
  cos(dz) : Trigonometry  Operator=cos
  dy= 90 : Constant  Value=90*d2r
  dz=0 : Constant  Value=0
  sin(dy) : Trigonometry
  sin(dz) : Trigonometry
  FL : Outport  InitialOutput=0
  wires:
  dz=0/1 -> sin(dz)/1, cos(dz)/1
  dy= 90/1 -> sin(dy)/1, cos(dy)/1
  sin(dy)/1 -> Fz1/2
  sin(dz)/1 -> Fy1/3
  cos(dz)/1 -> Fx1/3
  Mux/1 -> FL/1
  Fx1/1 -> Mux/1
  Fz1/1 -> Mux/3
  Fy1/1 -> Mux/2
  -1/1 -> Fz1/1
  cos(dy)/1 -> Fx1/2, Fy1/2
  Thrust/1 -> Fx1/1, Fy1/1, -1/1

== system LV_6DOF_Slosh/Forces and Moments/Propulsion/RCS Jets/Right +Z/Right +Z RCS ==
  note: Right +Z RCS Force
  Thrust : Inport
  -1 : Gain  Gain=-1
  Fx1 : Product  Inputs=3
  Fy1 : Product  Inputs=3
  Fz1 : Product
  Mux : Mux  Inputs=3
  cos(dy) : Trigonometry  Operator=cos
  cos(dz) : Trigonometry  Operator=cos
  dy=-90 : Constant  Value=-90*d2r
  dz=0 : Constant  Value=0
  sin(dy) : Trigonometry
  sin(dz) : Trigonometry
  FL : Outport  InitialOutput=0
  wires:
  dz=0/1 -> sin(dz)/1, cos(dz)/1
  dy=-90/1 -> sin(dy)/1, cos(dy)/1
  sin(dy)/1 -> Fz1/2
  sin(dz)/1 -> Fy1/3
  cos(dz)/1 -> Fx1/3
  Mux/1 -> FL/1
  Fx1/1 -> Mux/1
  Fz1/1 -> Mux/3
  Fy1/1 -> Mux/2
  -1/1 -> Fz1/1
  cos(dy)/1 -> Fx1/2, Fy1/2
  Thrust/1 -> Fx1/1, Fy1/1, -1/1

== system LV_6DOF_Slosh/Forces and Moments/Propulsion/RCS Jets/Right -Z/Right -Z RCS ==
  note: Right -Z RCS Force
  Thrust : Inport
  -1 : Gain  Gain=-1
  Fx1 : Product  Inputs=3
  Fy1 : Product  Inputs=3
  Fz1 : Product
  Mux : Mux  Inputs=3
  cos(dy) : Trigonometry  Operator=cos
  cos(dz) : Trigonometry  Operator=cos
  dy= 90 : Constant  Value=90*d2r
  dz=0 : Constant  Value=0
  sin(dy) : Trigonometry
  sin(dz) : Trigonometry
  FL : Outport  InitialOutput=0
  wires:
  dz=0/1 -> sin(dz)/1, cos(dz)/1
  dy= 90/1 -> sin(dy)/1, cos(dy)/1
  sin(dy)/1 -> Fz1/2
  sin(dz)/1 -> Fy1/3
  cos(dz)/1 -> Fx1/3
  Mux/1 -> FL/1
  Fx1/1 -> Mux/1
  Fz1/1 -> Mux/3
  Fy1/1 -> Mux/2
  -1/1 -> Fz1/1
  cos(dy)/1 -> Fx1/2, Fy1/2
  Thrust/1 -> Fx1/1, Fy1/1, -1/1

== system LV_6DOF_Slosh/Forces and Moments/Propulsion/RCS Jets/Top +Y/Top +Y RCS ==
  note: Top +Y RCS Force
  Thrust : Inport
  -1 : Gain  Gain=-1
  Fx1 : Product  Inputs=3
  Fy1 : Product  Inputs=3
  Fz1 : Product
  Mux : Mux  Inputs=3
  cos(dy) : Trigonometry  Operator=cos
  cos(dz) : Trigonometry  Operator=cos
  dy=0 : Constant  Value=0
  dz=+90 : Constant  Value=+90*d2r
  sin(dy) : Trigonometry
  sin(dz) : Trigonometry
  FL : Outport  InitialOutput=0
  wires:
  dz=+90/1 -> sin(dz)/1, cos(dz)/1
  dy=0/1 -> sin(dy)/1, cos(dy)/1
  sin(dy)/1 -> Fz1/2
  sin(dz)/1 -> Fy1/3
  cos(dz)/1 -> Fx1/3
  Mux/1 -> FL/1
  Fx1/1 -> Mux/1
  Fz1/1 -> Mux/3
  Fy1/1 -> Mux/2
  -1/1 -> Fz1/1
  cos(dy)/1 -> Fx1/2, Fy1/2
  Thrust/1 -> Fx1/1, Fy1/1, -1/1

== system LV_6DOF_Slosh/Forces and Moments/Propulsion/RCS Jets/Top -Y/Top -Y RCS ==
  note: Top -Y RCS Force
  Thrust : Inport
  -1 : Gain  Gain=-1
  Fx1 : Product  Inputs=3
  Fy1 : Product  Inputs=3
  Fz1 : Product
  Mux : Mux  Inputs=3
  cos(dy) : Trigonometry  Operator=cos
  cos(dz) : Trigonometry  Operator=cos
  dy=0 : Constant  Value=0
  dz=-90 : Constant  Value=-90*d2r
  sin(dy) : Trigonometry
  sin(dz) : Trigonometry
  FL : Outport  InitialOutput=0
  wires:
  dz=-90/1 -> sin(dz)/1, cos(dz)/1
  dy=0/1 -> sin(dy)/1, cos(dy)/1
  sin(dy)/1 -> Fz1/2
  sin(dz)/1 -> Fy1/3
  cos(dz)/1 -> Fx1/3
  Mux/1 -> FL/1
  Fx1/1 -> Mux/1
  Fz1/1 -> Mux/3
  Fy1/1 -> Mux/2
  -1/1 -> Fz1/1
  cos(dy)/1 -> Fx1/2, Fy1/2
  Thrust/1 -> Fx1/1, Fy1/1, -1/1

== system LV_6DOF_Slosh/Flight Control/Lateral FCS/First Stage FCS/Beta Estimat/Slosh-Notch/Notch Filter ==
  note: Variable Notch Filter
  u : Inport
  2.z1.w : Subsystem
  2.z2.w : Subsystem
  Sum1 : Sum  Inputs=+++
  Sum3 : Sum  Inputs=+--
  int{1..4} (4 alike) : Integrator
  w^2 : Subsystem
  "w^2 " : Subsystem
  y : Outport
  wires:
  u/1 -> Sum1/1, int1/1
  int2/1 -> "w^2 "/1(in)
  int1/1 -> 2.z1.w/1(in), int2/1
  int3/1 -> 2.z2.w/1(in), int4/1
  Sum1/1 -> Sum3/1
  Sum3/1 -> y/1, int3/1
  2.z2.w/1(ou) -> Sum3/3
  int4/1 -> w^2/1(in)
  "w^2 "/1(ou) -> Sum1/3
  w^2/1(ou) -> Sum3/2
  2.z1.w/1(ou) -> Sum1/2

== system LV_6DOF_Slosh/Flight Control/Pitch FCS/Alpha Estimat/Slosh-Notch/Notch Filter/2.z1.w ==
  in : Inport
  2.z1.w : Gain  Gain=0.016
  Product1 : Product
  ou : Outport
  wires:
  2.z1.w/1 -> Product1/1
  Product1/1 -> ou/1
  in/1 -> Product1/2
  [Wnf] -> 2.z1.w/1

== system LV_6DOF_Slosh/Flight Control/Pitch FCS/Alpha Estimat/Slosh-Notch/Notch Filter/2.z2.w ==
  in : Inport
  2.z2.w : Gain  Gain=0.32
  Product1 : Product
  ou : Outport
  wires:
  2.z2.w/1 -> Product1/1
  Product1/1 -> ou/1
  in/1 -> Product1/2
  [Wnf] -> 2.z2.w/1

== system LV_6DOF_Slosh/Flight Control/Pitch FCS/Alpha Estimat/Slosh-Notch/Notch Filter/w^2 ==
  in : Inport
  Product : Product
  Product1 : Product
  ou : Outport
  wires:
  [Wnf] -> Product/1, Product/2
  Product/1 -> Product1/1
  Product1/1 -> ou/1
  in/1 -> Product1/2

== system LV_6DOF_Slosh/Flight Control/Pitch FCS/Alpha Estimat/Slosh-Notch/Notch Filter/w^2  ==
  in : Inport
  Product : Product
  Product1 : Product
  ou : Outport
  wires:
  [Wnf] -> Product/1, Product/2
  Product/1 -> Product1/1
  Product1/1 -> ou/1
  in/1 -> Product1/2

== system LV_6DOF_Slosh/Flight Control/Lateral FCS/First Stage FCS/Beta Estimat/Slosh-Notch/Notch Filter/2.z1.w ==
  in : Inport
  2.z1.w : Gain  Gain=0.016
  Product1 : Product
  ou : Outport
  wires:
  2.z1.w/1 -> Product1/1
  Product1/1 -> ou/1
  in/1 -> Product1/2
  [Wnf] -> 2.z1.w/1

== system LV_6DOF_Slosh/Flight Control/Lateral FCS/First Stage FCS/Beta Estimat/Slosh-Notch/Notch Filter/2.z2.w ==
  in : Inport
  2.z2.w : Gain  Gain=0.32
  Product1 : Product
  ou : Outport
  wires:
  2.z2.w/1 -> Product1/1
  Product1/1 -> ou/1
  in/1 -> Product1/2
  [Wnf] -> 2.z2.w/1

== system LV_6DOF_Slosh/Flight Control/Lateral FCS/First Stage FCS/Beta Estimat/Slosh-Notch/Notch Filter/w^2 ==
  in : Inport
  Product : Product
  Product1 : Product
  ou : Outport
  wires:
  [Wnf] -> Product/1, Product/2
  Product/1 -> Product1/1
  Product1/1 -> ou/1
  in/1 -> Product1/2

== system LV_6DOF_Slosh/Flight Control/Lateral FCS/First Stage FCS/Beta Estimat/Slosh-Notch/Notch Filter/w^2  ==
  in : Inport
  Product : Product
  Product1 : Product
  ou : Outport
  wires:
  [Wnf] -> Product/1, Product/2
  Product/1 -> Product1/1
  Product1/1 -> ou/1
  in/1 -> Product1/2

== matlab function LV_6DOF_Slosh/Flight Control/Commands/Quaternion Error
Function ==
function qfb = Qerror(qc,qb)
% Calculates the Quaternion error vector in (radians)
% used for Attitude Feedback
% [qfb]= Qerror(qd,qb);
[qfb]=qerang( qmult6dof2(1,0,qb,qc) );
end

function [q3]=qmult6dof2(n1,n2,q1,q2)
q1v=zeros(1,3); q2v=q1v; q1d=q1v; q2d=q1v; q3=zeros(1,4);
q1s=q1(1); q2s=q2(1);
for  i=1:3
    q1v(i)=q1(i+1);
    q2v(i)=q2(i+1);
end
%     N1 <> 1 ===> TAKE CONJUGATE OF Q1V
%     N2 <> 1 ===> TAKE CONJUGATE OF Q2V
for  i=1:3
    q1d(i)=q1v(i);
    q2d(i)=q2v(i);
    if(n1 ~= 1)
        q1d(i)=-q1v(i);
    end
    if(n2 ~= 1)
        q2d(i)=-q2v(i);
    end
end
q3(1)=q1s.*q2s-(q1d(1).*q2d(1)+q1d(2).*q2d(2)+q1d(3).*q2d(3));
q3(2)=q1s.*q2d(1)+q2s.*q1d(1)+q1d(2).*q2d(3)-q1d(3).*q2d(2);
q3(3)=q1s.*q2d(2)+q2s.*q1d(2)-q1d(1).*q2d(3)+q1d(3).*q2d(1);
q3(4)=q1s.*q2d(3)+q2s.*q1d(3)+q1d(1).*q2d(2)-q1d(2).*q2d(1);
end

function [eba]=qerang(qba)      %  Quatern_Error Angle
qbas=qba(1);
qbav=zeros(1,3);
for  i=1:3; qbav(i)=qba(i+1); end
temp= sign1(qbas);
atterr=-2.*temp;
eba=atterr.*qbav;
end

function s=sign1(v)
s=sign(v);
if (s==0); s=1.; end
end

== matlab function LV_6DOF_Slosh/Flight Control/RCS Control/Phase-Plane
Controller/MATLAB Function ==
function [fp,eu,Isel]= Phase_Plane(Rater,Atter, J11,J22,J33,Xcg,Jdir,Jloc)    
% Phase-Plane Logic for RCS jets
% Rater: Rate Error in (deg/sec)
% Atter: Attitude Error in (deg)

% Define Phase-Plane Logic Parameters in (deg)
r2d=180/pi;
Thr=3.0 ;                                               % Thrust (lb)
nt=8;                                                   % Number of Jets
cg2= [Xcg, 0.0, 0.0]';                                  % CG Location
ang_acl     = Thr*[6/J11, 20/J22, 20/J33]*10;
att_deadband= [1, 1, 1]*0.25;
kledge      = [1.2,  1.2,  1.2];
rate_lim    = [1, 1, 1]*4.0; 
low_rate_lim= rate_lim*0.32;

rat_err= -Rater*r2d;                                    % Convert to (deg)
att_err= -Atter*r2d;
Cnt= [0;0;0];                                           % Control to JetSel

for iax=1:3
    sign_rat_err= sign(rat_err(iax)+1.0e-8);
    x1 = sign_rat_err*att_err(iax);
    x2 = abs(rat_err(iax));
    ang_acl_gain= 2*ang_acl(iax);
    curve = rat_err(iax)^2/ang_acl_gain;
    
    sw1= -curve + att_deadband(iax);
    sw2= -(curve + (kledge(iax)*att_deadband(iax)));
    sw3= rate_lim(iax);
    sw5= low_rate_lim(iax);
    
    if (x1>sw1) || (x2>sw3), Cnt(iax)= -sign_rat_err;   % Region 1
    elseif (x1 >= sw2), Cnt(iax)= 0;                    % Region 2
    elseif (x2 < sw5), Cnt(iax)= sign_rat_err;          % Region 3
    else, Cnt(iax)= 0;  
    end
end

% Select Jets and Calculate Rotation Vector
Mg=sqrt(Cnt'*Cnt);
if Mg>0
    eu= Cnt/Mg;                                         % Rotation Vector
    [fp,Isel]= Jet_Select_dot(-eu,4, nt,Thr,cg2,Jloc,Jdir); % Thruster Forces
else
    eu= Cnt; fp=zeros(nt,1); Isel=0;                    % No Firing
end


function [fp,Isel]= Jet_Select_dot(eu,Imax, nt,Thr,cg2,Jloc,Jdir)
% fp= Jet_Select_dot(eu,nt,Thr,Jloc,Jdir,Imax)
% Compute the thrust force vector (fp)
% Inputs
% eu(3) : ACS error unit vector
% nt    : number of jets
% Thr   : Thrust in (lb)
% Jloc  : Jet Locations 
% Jdir  : Thrust directions
% Imax  : Max number of Thrusters to select
% J     : Vehicle MOI matrix (3x3)
% cg(3) : CG location
% Outputs
% fp(nt): Thrusts vector (nt)

if sqrt(eu'*eu)<0.9                                 % Direction must be unit vect
    fp=zeros(nt,1); Isel=0; return; 
end    

tm= Thr*ones(1,nt);
vt= zeros(3,nt); ln=vt; 
pf= zeros(nt,1); sf=pf;

% Select the most dominant jets from all of them
for i=1:nt
    ln(:,i)= Jloc(:,i) - cg2;                       % Moment arms
    vt(:,i)= tm(i)*cross(ln(:,i),Jdir(:,i));        % Moments Matrix using all jets
    pf(i) = dot(vt(:,i),eu);                        % Moment dotted with maneuv direct
end

f2=pf;
for i=1:(nt/2)
    [mf,sf(i)]=max(f2); f2(sf(i))=0;                % Identify the strongest half
end
pf= pf/pf(sf(1));                                   % Normlz relative to strongest

% Select Imax jets among the strongest
Isel=1;                                             % First, select the strongest
for i=1:Imax-1
    if pf(sf(i+1))>0.72; Isel=Isel+1; end            % 70% contrib, choose one more jet to Imax
end

fp= zeros(nt,1);                                    % Initially zero all jets
for i=1:nt
    for j=1:Isel
        if i==sf(j); fp(i)=Thr; end                 % Turn on the selected jet force
    end
end

== matlab function LV_6DOF_Slosh/Vehicle 6-DOF/Rate Gyros/Quaternion 
Derivative ==
function Qd=Qtdot(qi,wb)
%  THIS SUBROUTINE FINDS THE DERIVATIVES A,
%   OF QUATERNION qi, SUBJECT TO ANGULAR RATES Wb;
d= [0.0, -0.5*wb(1), -0.5*wb(2), -0.5*wb(3)];
[Qd]=qmult6dof(1,1,d,qi);
%
function [q3]=qmult6dof(n1,n2,q1,q2)
q1v=zeros(1,3); q2v=q1v; q1d=q1v; q2d=q1v; q3=zeros(1,4);
q1s=q1(1); q2s=q2(1);

for  i=1:3
    q1v(i)=q1(i+1);
    q2v(i)=q2(i+1);
end
%     N1 <> 1 ===> TAKE CONJUGATE OF Q1V
%     N2 <> 1 ===> TAKE CONJUGATE OF Q2V
for  i=1:3
    q1d(i)=q1v(i);
    q2d(i)=q2v(i);
    if(n1 ~= 1)
        q1d(i)=-q1v(i);
    end
    if(n2 ~= 1)
        q2d(i)=-q2v(i);
    end
end
q3(1)=q1s.*q2s-(q1d(1).*q2d(1)+q1d(2).*q2d(2)+q1d(3).*q2d(3));
q3(2)=q1s.*q2d(1)+q2s.*q1d(1)+q1d(2).*q2d(3)-q1d(3).*q2d(2);
q3(3)=q1s.*q2d(2)+q2s.*q1d(2)-q1d(1).*q2d(3)+q1d(3).*q2d(1);
q3(4)=q1s.*q2d(3)+q2s.*q1d(3)+q1d(1).*q2d(2)-q1d(2).*q2d(1);

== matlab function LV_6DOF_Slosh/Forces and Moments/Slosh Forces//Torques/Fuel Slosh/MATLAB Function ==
function [xdot,u1,u2,Fv,delta,Wsl,theta]= Slosh(x,Acc,Msl,Rsl,Zeta) 
% Slosh Model  
% out= Slosh(x,Acc)  
% Calculates the Slosh Forces on the Tank as a function of 
% Vehicle acceleration at the Tank
%
% State Variables (x) 
% x(1:3)  = Xsd Slosh Mass Velocity wrt Tank 
% x(4:6)  = Xs Slosh Mass Position wrt Tank 
% Acc(3}  = Vehicle Linear x,y,z Accelerat at Tank
% Msl     = Slosh Mass (slug)
% Rsl     = Pendulum length (ft)
% Ts      = Sampling Period (sec)

xdot=zeros(6,1);                                      % Initialize
Xsd= x(1:3);                                          % Velocity of Msl (Tank Relative)
Xs = x(4:6);                                          % Position of Msl (Tank Relative)

% Find the Axial direction u1
rs= sqrt(Xs'*Xs);                                     % Scalar Distance of Msl from center
if rs==0, rs=0.0001;                                  % Avoid Xs in the center of sphere
    e=rand(3,1); Xs=e*rs/sqrt(e'*e);
end
u1= Xs/rs;                                            % Unit vector from center to mass
theta=acos(-u1(1));                                   % Pendulum Angle wrt tank centerline

% Find the Tangential direction u2 
vm= sqrt(Xsd'*Xsd);                                   % Veloc magnit relative to tank
if vm==0, vm=0.0001;                                  % Avoid Xsd being zero
    e=rand(3,1); Xsd=e*vm/sqrt(e'*e);
end
uv= Xsd/vm;                                           % Unit vector along veloc Xsd
u3= cross(u1,uv);                                     % Unit Vect Perpendic to u1 & uv
u2= cross(u3,u1);                                     % Unit Vect along vel, Tangent to surface

% Non-Linear Spring Deflection 
delta= rs - Rsl;                                      % Spring Extension
if delta>0                                            % Stretched Spring
    Kspr=(8000*delta^2 + 100)*Msl;                    % Non-Linear Spring 2.e5*delta^2 + 5.0e3;
    Kd1=2+8*Msl;                                      % Friction Coefficients 1000
    Wsl= dot((Xsd/rs),u2);                            % Slosh Mass angular rate tangent tank surf
    if Acc(1)>0
          Kfr=2*Msl*Zeta*sqrt(Acc(1)*Rsl);            % Friction Coefficient
    else, Kfr=0; 
    end
else                                                  % Free-Floating
    Kspr=0; Kfr=0; Kd1=0; Wsl=0; delta=0;             % Zero all External Forces
end

% Forces on Slosh Mass and Vehicle 
Fd= Kfr*Wsl;                                          % Tangent Viscous Frict Force on Mass
Fst= Kspr*delta + Msl*(rs*Wsl^2) + dot(Kd1*Xsd,u1);   % Radial Centripet, Spring & Dampinq accel
Xsdd= - (Fst/Msl)*u1 - (Fd/Msl)*u2 - Acc;             % Slosh mass Acceler wrt tank center
Fv= Fst*u1 + Fd*u2; Fv(1)=0;                          % Y,Z Force on Vehicle, No X

% State Derivatives 
xdot(1:3)= Xsdd;                                      % Xs-dot-dot 
xdot(4:6)= Xsd;                                       % Xs-dot 
end

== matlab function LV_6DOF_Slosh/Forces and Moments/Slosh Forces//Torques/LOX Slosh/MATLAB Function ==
function [xdot,u1,u2,Fv,delta,Wsl,theta]= Slosh(x,Acc,Msl,Rsl,Zeta) 
% Slosh Model  
% out= Slosh(x,Acc)  
% Calculates the Slosh Forces on the Tank as a function of 
% Vehicle acceleration at the Tank
%
% State Variables (x) 
% x(1:3)  = Xsd Slosh Mass Velocity wrt Tank 
% x(4:6)  = Xs Slosh Mass Position wrt Tank 
% Acc(3}  = Vehicle Linear x,y,z Accelerat at Tank
% Msl     = Slosh Mass (slug)
% Rsl     = Pendulum length (ft)
% Ts      = Sampling Period (sec)

xdot=zeros(6,1);                                      % Initialize
Xsd= x(1:3);                                          % Velocity of Msl (Tank Relative)
Xs = x(4:6);                                          % Position of Msl (Tank Relative)

% Find the Axial direction u1
rs= sqrt(Xs'*Xs);                                     % Scalar Distance of Msl from center
if rs==0, rs=0.0001;                                  % Avoid Xs in the center of sphere
    e=rand(3,1); Xs=e*rs/sqrt(e'*e);
end
u1= Xs/rs;                                            % Unit vector from center to mass
theta=acos(-u1(1));                                   % Pendulum Angle wrt tank centerline

% Find the Tangential direction u2 
vm= sqrt(Xsd'*Xsd);                                   % Veloc magnit relative to tank
if vm==0, vm=0.0001;                                  % Avoid Xsd being zero
    e=rand(3,1); Xsd=e*vm/sqrt(e'*e);
end
uv= Xsd/vm;                                           % Unit vector along veloc Xsd
u3= cross(u1,uv);                                     % Unit Vect Perpendic to u1 & uv
u2= cross(u3,u1);                                     % Unit Vect along vel, Tangent to surface

% Non-Linear Spring Deflection 
delta= rs - Rsl;                                      % Spring Extension
if delta>0                                            % Stretched Spring
    Kspr=(8000*delta^2 + 100)*Msl;                    % Non-Linear Spring 2.e5*delta^2 + 5.0e3;
    Kd1=2+8*Msl;                                      % Friction Coefficients 1000
    Wsl= dot((Xsd/rs),u2);                            % Slosh Mass angular rate tangent tank surf
    if Acc(1)>0
          Kfr=2*Msl*Zeta*sqrt(Acc(1)*Rsl);            % Friction Coefficient
    else, Kfr=0; 
    end
else                                                  % Free-Floating
    Kspr=0; Kfr=0; Kd1=0; Wsl=0; delta=0;             % Zero all External Forces
end

% Forces on Slosh Mass and Vehicle 
Fd= Kfr*Wsl;                                          % Tangent Viscous Frict Force on Mass
Fst= Kspr*delta + Msl*(rs*Wsl^2) + dot(Kd1*Xsd,u1);   % Radial Centripet, Spring & Dampinq accel
Xsdd= - (Fst/Msl)*u1 - (Fd/Msl)*u2 - Acc;             % Slosh mass Acceler wrt tank center
Fv= Fst*u1 + Fd*u2; Fv(1)=0;                          % Y,Z Force on Vehicle, No X

% State Derivatives 
xdot(1:3)= Xsdd;                                      % Xs-dot-dot 
xdot(4:6)= Xsd;                                       % Xs-dot 
end
